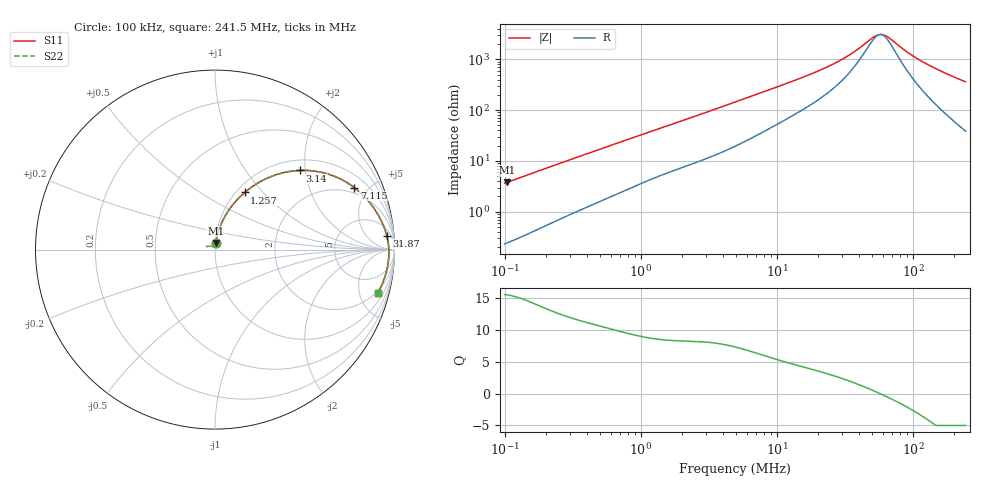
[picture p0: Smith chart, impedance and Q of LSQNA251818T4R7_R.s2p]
! LSQNA251818T4R7_R  S-PARAMETER MODEL  ( General Type )
! Model Generated by TAIYO YUDEN Corporation (http://www.ty-top.com)
! Version 2.0
! TAIYO YUDEN Control No. 100810NF25SB-FKC
! Copyright(c) 2007 TAIYO YUDEN CO.,LTD. All Rights Reserved.
! Product Description (link to TY-COMPAS)
! https://ds.yuden.co.jp/TYCOMPAS/or/detail?pn=LSQNA251818T4R7MR&u=M
! Products Name : Inductors
! Characteristics :
!  Inductance : 4.7 uH , SRF(min) : 46 MHz , DC Resistance(max) : 0.13 Ohm
!  Rated Current : Saturation :310 mA , Temp Rise : 1200 mA (40 degC)
!  Case Size : 2.5 x 1.8 / 0.098 x 0.071 [mm/inch] , Thickness : 1.8 / 0.071 [mm/inch]
!  (Conditions: Temperature = 25 degC , DC Bias Current/Voltage = 0A / 0V)
! External Node Assignments :
!  1  o---GGG---o  2
! GND o---------o GND
! Frequency Range : 0.1MHz  -  241.513628MHz  [ 402 STEP ]
# MHz S RI R 50
! Freq[MHz].  S11 Real  S11 Imag  S21 Real  S21 Imag  S12 Real  S12 Imag  S22 Real  S22 Imag
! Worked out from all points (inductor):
!   401 points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, 100 kHz to 241.5 MHz, reference 50 ohm
!   read as one part in series: L = 5.74 uH near 104 kHz
!   highest Q = 15.6 at 104 kHz (marker M1), where L = 5.77 uH
!   self-resonance near 57.22 MHz
!   S11 on the Smith chart (normalised r, x): 100 kHz: 1.00, +0.07; 1.257 MHz: 1.09, +0.80; 3.14 MHz: 1.23, +1.87; 7.115 MHz: 1.64, +4.07; 31.87 MHz: 10, +20; 241.5 MHz: 1.78, -7.19
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0.1  0.00362 0.036  0.9964 -0.036  0.9964 -0.036  0.00362 0.036
0.103972  0.00382 0.0374  0.9962 -0.0374  0.9962 -0.0374  0.00382 0.0374
0.205552  0.0107 0.0718  0.9893 -0.0718  0.9893 -0.0718  0.0107 0.0718
0.368674  0.0264 0.1223  0.9736 -0.1223  0.9736 -0.1223  0.0264 0.1223
0.72887  0.0754 0.2175  0.9246 -0.2175  0.9246 -0.2175  0.0754 0.2175
1.25735  0.1655 0.3183  0.8345 -0.3183  0.8345 -0.3183  0.1655 0.3183
1.359207  0.1837 0.3331  0.8163 -0.3331  0.8163 -0.3331  0.1837 0.3331
2.006469  0.298 0.401  0.702 -0.401  0.702 -0.401  0.298 0.401
3.140159  0.4727 0.4412  0.5273 -0.4412  0.5273 -0.4412  0.4727 0.4412
4.914404  0.6557 0.412  0.3443 -0.412  0.3443 -0.412  0.6557 0.412
7.114765  0.7756 0.3459  0.2244 -0.3459  0.2244 -0.3459  0.7756 0.3459
10.91999  0.8662 0.2566  0.1338 -0.2566  0.1338 -0.2566  0.8662 0.2566
18.11814  0.9256 0.1624  0.0744 -0.1624  0.0744 -0.1624  0.9256 0.1624
24.74179  0.9465 0.113  0.0535 -0.113  0.0535 -0.113  0.9465 0.113
31.86961  0.9575 0.0767  0.0425 -0.0767  0.0425 -0.0767  0.9575 0.0767
53.91696  0.9683 0.00762  0.0317 -0.00762  0.0317 -0.00762  0.9683 0.00762
59.43088  0.9688 -0.00486  0.0312 0.00486  0.0312 0.00486  0.9688 -0.00486
66.79689  0.9689 -0.02  0.0311 0.02  0.0311 0.02  0.9689 -0.02
89.45746  0.9666 -0.0595  0.0334 0.0595  0.0334 0.0595  0.9666 -0.0595
115.2291  0.9608 -0.0974  0.0392 0.0974  0.0392 0.0974  0.9608 -0.0974
163.6042  0.9444 -0.1586  0.0556 0.1586  0.0556 0.1586  0.9444 -0.1586
241.5136  0.9066 -0.242  0.0934 0.242  0.0934 0.242  0.9066 -0.242
